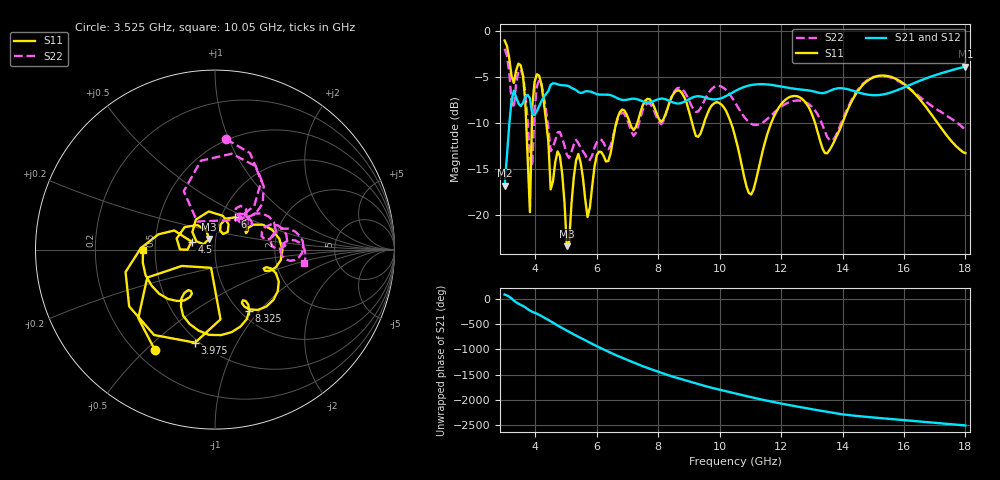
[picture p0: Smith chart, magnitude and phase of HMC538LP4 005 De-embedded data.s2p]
! Chelmsford, MA 01824
! http://www.hittite.com
! Tel: 978-250-3343
! Fax: 978-250-3373
! Device  :  HMC538LP4
! Description:  600 Analog Phase Shifter
! Frequency  :  6.0 GHz - 15.0 GHz
! Package  :  LP4  - 4x4 mm Quad Flatpack No-Lead (QFN) Plastic Package: 24 pin
! Ports  :  2 RF, 1 DC
!  Pin  3  = Rfin  = Port 1
!  Pin  16  = Rfout = Port 2
!  pin  21  = vCTL
! Voltages:  VCTL  = 0 to 5.0 Volts
! Currents :  Vb(V)  Vd(V)  Ib(mA)  Id(mA)
!  0.00  0.50  0.000000	0.483019
! Data:  The device was measured on evaluation board 111296-1.
!  Data was collected using a calibrated network analyzer.
!  The evaluation circuit board was modeled and simulated.This was use
!  to removed the evaluation board circuit from the measured data.
!  The reference plane is the center of the package pin.
! Misc:  Lot #
!Date Measured:  03 - 11 -2009
! Date:  03 - 17 -2009
! Note:
!  Hittite Microwave supplies this data as a sample of measured data at the
!  package pin for this package product.  Your particular data for this product
!  may vary.
!  Data was taken at 25 degrees C.
!  Hittite Microwave reserves the right to change this data at anytime.
# MHz S MA R 50
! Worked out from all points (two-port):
!   201 points, 3 GHz to 18 GHz, reference 50 ohm
!   highest |S21| = -3.83 dB at 18 GHz (marker M1); lowest = -16.8 dB at 3 GHz (marker M2)
!   |S21| within 3 dB of the highest: 10.33 GHz to 14.73 GHz (4.402 GHz wide, 35.1 % of centre); 15.38 GHz to end of sweep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
!   lowest |S11| = -23.4 dB at 5.025 GHz (marker M3), VSWR 1.15, Z = 46.6 + j5.61 ohm
!   |S11| at or under -10 dB: 4.359 GHz to 6.633 GHz (2.273 GHz wide, 41.4 % of centre); 10.37 GHz to 11.68 GHz (1.302 GHz wide, 11.8 % of centre); 13.11 GHz to 13.99 GHz (882.6 MHz wide, 6.51 % of centre)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
!   |S22| runs from -14.7 to -1.9 dB; largest |S21 - S12| = 0.0018
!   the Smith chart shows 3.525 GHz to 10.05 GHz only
!   S11 on the Smith chart (normalised r, x): 3.525 GHz: 0.27, -0.54; 3.975 GHz: 0.48, -0.69; 4.5 GHz: 0.77, +0.07; 6 GHz: 1.17, +0.44; 8.325 GHz: 1.10, -0.88; 10.05 GHz: 0.43, -0.00
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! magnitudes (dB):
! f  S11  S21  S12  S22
! 3 GHz  -1.0  -16.8  -16.8  -1.9
! 3.225 GHz  -4.9  -7.5  -7.5  -7.5
! 3.525 GHz  -3.7  -8.1  -8.1  -4.2
! 3.825 GHz  -19.7  -7.3  -7.3  -13.8
! 3.975 GHz  -5.5  -9.1  -9.1  -8.7
! 4.2 GHz  -5.8  -7.6  -7.6  -5.7
! 4.5 GHz  -17.2  -5.8  -5.8  -13.0
! 4.8 GHz  -13.5  -5.8  -5.8  -10.9
! 5.025 GHz  -23.4  -5.9  -5.9  -13.4
! 5.325 GHz  -14.1  -6.4  -6.4  -11.8
! 5.55 GHz  -15.9  -6.7  -6.7  -13.0
! 5.7 GHz  -20.2  -6.5  -6.5  -14.0
! 6 GHz  -13.5  -6.8  -6.8  -12.1
! 8.025 GHz  -9.5  -7.4  -7.4  -9.9
! 8.325 GHz  -8.2  -7.5  -7.5  -8.2
! 10.05 GHz  -7.9  -7.3  -7.3  -6.0
! 10.5 GHz  -11.4  -6.5  -6.5  -7.7
! 11.03 GHz  -17.7  -5.8  -5.8  -10.0
! 12 GHz  -7.9  -6.0  -6.0  -8.2
! 13.05 GHz  -9.4  -6.5  -6.5  -8.4
! 15.53 GHz  -4.9  -6.7  -6.7  -5.0
! 18 GHz  -13.2  -3.8  -3.8  -10.7
